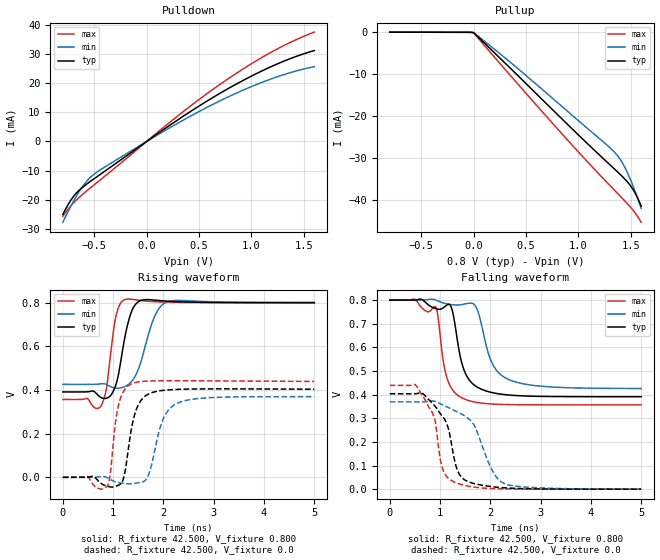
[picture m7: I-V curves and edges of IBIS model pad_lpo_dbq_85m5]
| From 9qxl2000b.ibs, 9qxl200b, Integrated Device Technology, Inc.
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|   Model pad_lpo_dbq_85m5
[Model] pad_lpo_dbq_85m5
Model_type Output
Polarity   Non-Inverting
Vmeas =  0.200V
Cref =  0.0F
Rref =  42.500
Vref =  0.350V
C_comp   1.000fF   1.000fF   1.000fF
[Temperature Range]   65.000   0.125k   -10.000
[Voltage Range]   0.800V   0.800V   0.800V
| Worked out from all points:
|   slope of the pulldown table from 0 to 0.12 V, typ, clamps not added: 39.3 ohm
|   slope of the pullup table from 0 to 0.12 V, typ, clamps not added: 41.6 ohm
|   rising waveform, R_fixture 42.500, V_fixture 0.800: 20-80 % time 202ps typ, 293ps min, 144ps max; typ from 0.392 V to 0.801 V
|   rising waveform, R_fixture 42.500, V_fixture 0.0: 20-80 % time 209ps typ, 280ps min, 156ps max; typ from 0 V to 0.404 V
|   falling waveform, R_fixture 42.500, V_fixture 0.800: 20-80 % time 267ps typ, 340ps min, 211ps max; typ from 0.801 V to 0.392 V
|   falling waveform, R_fixture 42.500, V_fixture 0.0: 20-80 % time 352ps typ, 473ps min, 284ps max; typ from 0.404 V to 0 V
[Pulldown]
|Voltage   I(typ)   I(min)   I(max)
-800mV    -25.03mA   -27.67mA   -25.65mA
-750mV    -21.65mA   -24.02mA   -23.18mA
-700mV    -18.92mA   -20.61mA   -21.1mA
-600mV    -15.37mA   -14.85mA   -17.78mA
-525mV    -13.38mA   -11.92mA   -15.57mA
-375mV    -9.575mA   -8.217mA   -11.2mA
275mV     6.848mA    5.788mA    8.108mA
725mV     17mA       14.34mA    20.16mA
975mV     21.91mA    18.4mA     26.04mA
1.2V      25.8mA     21.55mA    30.78mA
1.4V      28.76mA    23.86mA    34.4mA
1.6V      31.11mA    25.6mA     37.44mA
[Pullup]
|Voltage   I(typ)   I(min)   I(max)
-800mV    81.85uA    71.33uA    95.65uA
0V        -29.45uA   -29.07uA   -41.09uA
350mV     -8.476mA   -7.071mA   -10.18mA
750mV     -18.28mA   -15.59mA   -21.51mA
1.075V    -26.17mA   -22.58mA   -30.45mA
1.275V    -30.88mA   -26.84mA   -35.74mA
1.35V     -32.63mA   -28.63mA   -37.68mA
1.425V    -34.42mA   -31.23mA   -39.61mA
1.475V    -35.76mA   -33.73mA   -40.94mA
1.525V    -37.47mA   -36.73mA   -42.41mA
1.55V     -38.57mA   -38.38mA   -43.24mA
1.6V      -41.37mA   -41.89mA   -45.18mA
[Ramp]
| variable   typ   min   max
dV/dt_r   0.242/0.210n   0.222/0.281n   0.264/0.156n
dV/dt_f   0.246/0.269n   0.225/0.346n   0.266/0.212n
R_load = 42.500
[Rising Waveform]
R_fixture= 42.500
V_fixture= 0.800
V_fixture_min= 0.800
V_fixture_max= 0.800
|time   V(typ)   V(min)   V(max)
0s        391.5mV    426.2mV    357mV
765ps     364.9mV    429mV      330mV
863ps     362.5mV    426mV      403.2mV
1.033ns   410.9mV    409.3mV    710.8mV
1.234ns   643.8mV    416.6mV    815.1mV
1.347ns   748mV      434.6mV    816.7mV
1.476ns   800.6mV    481.8mV    812.9mV
1.81ns    812.8mV    729.6mV    805.5mV
2.08ns    807.7mV    805mV      803.1mV
5ns       800.7mV    800.9mV    800.8mV
[Rising Waveform]
R_fixture= 42.500
V_fixture= 0.0
V_fixture_min= 0.0
V_fixture_max= 0.0
|time   V(typ)   V(min)   V(max)
0s        13.51uV    129.6uV    9.707uV
877ps     -40.66mV   -923.2uV   -42.24mV
936ps     -43.67mV   -8.72mV    4.901mV
1.107ns   -35.98mV   -24.21mV   330.4mV
1.228ns   16.65mV    -28.3mV    402mV
1.382ns   244.5mV    -29.21mV   430.3mV
1.678ns   378.7mV    -1.049mV   441.1mV
1.982ns   398.4mV    260mV      442.7mV
2.262ns   403mV      338.2mV    442.8mV
5ns       404.1mV    369.7mV    439.6mV
[Falling Waveform]
R_fixture= 42.500
V_fixture= 0.800
V_fixture_min= 0.800
V_fixture_max= 0.800
|time   V(typ)   V(min)   V(max)
0s        800.7mV    800.9mV    800.9mV
913ps     764.8mV    801.2mV    771.5mV
963ps     761.9mV    797mV      726mV
1.073ns   769.5mV    788.1mV    532mV
1.214ns   774.9mV    782.1mV    432.4mV
1.482ns   501.8mV    784mV      382mV
1.713ns   435.9mV    772.6mV    367.9mV
2.026ns   409.5mV    537.9mV    360.7mV
2.376ns   398.6mV    463.2mV    358.1mV
5ns       391.5mV    426.2mV    357mV
[Falling Waveform]
R_fixture= 42.500
V_fixture= 0.0
V_fixture_min= 0.0
V_fixture_max= 0.0
|time   V(typ)   V(min)   V(max)
0s        404.1mV    369.7mV    439.6mV
555ps     405.4mV    369.4mV    429.7mV
882ps     356mV      372.8mV    305mV
1.011ns   318.1mV    361.1mV    119.5mV
1.102ns   292mV      351.7mV    62.66mV
1.292ns   119.8mV    332.5mV    29.51mV
1.671ns   24.09mV    273.6mV    8.977mV
2.022ns   10.94mV    86.08mV    2.734mV
2.26ns    6.119mV    25.16mV    1.208mV
5ns       13.53uV    130uV      9.706uV
